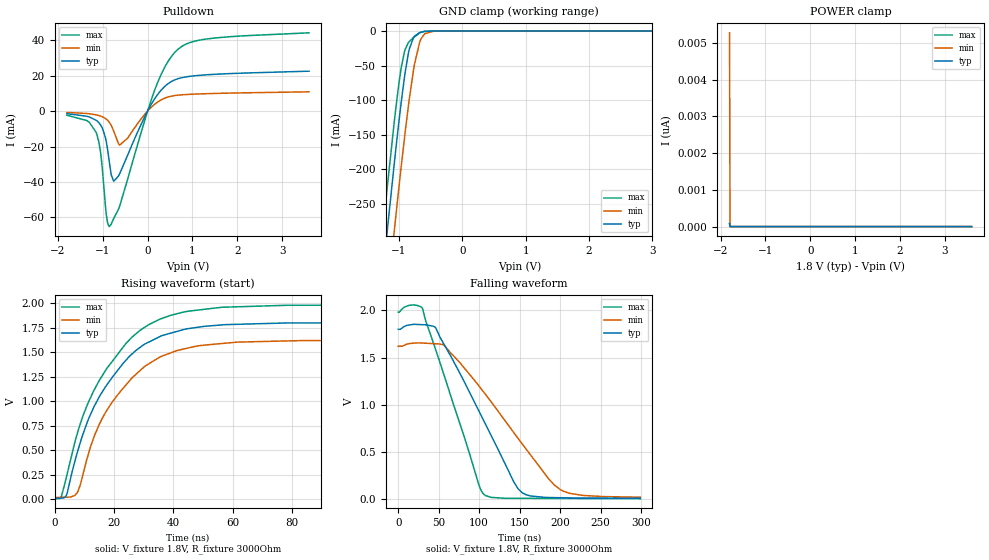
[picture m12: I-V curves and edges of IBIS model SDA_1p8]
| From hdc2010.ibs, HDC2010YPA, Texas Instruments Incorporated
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[Model]   SDA_1p8
Model_type   I/O_open_drain
Polarity   Non-Inverting
Enable   Active-Low
Vinl = 0.54
Vinh = 1.26
Vmeas = 0.9
Vref = 1.8
Cref = 15pF
Rref = 3000
|   typ   min   max
|   (nom PVT)   (slow PVT)   (fast PVT)
C_comp   1.615p   1.567p   1.665p
|C_comp (ON state)   1.615p   1.567p   1.665p
|C_comp (OFF state)   1.693p   1.643p   1.788p
[Model spec]
|subparameter
Vinl   0.54   0.486   0.594
Vinh   1.26   1.134   1.386
[Voltage Range]   1.8   1.62   1.98
[Temperature Range]   27   125   -40
[Pullup Reference]   1.8   1.62   1.98
[Pulldown Reference]   0   -0   0
[Power Clamp Reference]   1.8   1.62   1.98
[GND Clamp Reference]   0   0   0
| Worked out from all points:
|   slope of the pulldown table from 0 to 0.27 V, typ, clamps not added: 24.9 ohm
|   GND clamp passes 1 mA (typ) near -0.62 V on its own axis
|   falling waveform, V_fixture 1.8V, R_fixture 3000Ohm: 20-80 % time 62.9ns typ, 84.5ns min, 44.7ns max; typ from 1.8 V to 0.012 V
|   rising waveform, V_fixture 1.8V, R_fixture 3000Ohm: 20-80 % time 18.1ns typ, 18.1ns min, 18.6ns max; typ from 0.012 V to 1.8 V
[Pulldown]
|   Voltage   I(typ)   I(min)   I(max)
-1.8V     -1.437mA   -727.9uA   -2.321mA
-1.357V   -2.889mA   -1.337mA   -5.326mA
-1.147V   -5.182mA   -2.104mA   -12.02mA
-1.044V   -7.982mA   -2.835mA   -24.2mA
-941.4mV  -14.84mA   -4.15mA    -53.24mA
-855mV    -28.46mA   -6.275mA   -65.18mA
-757.8mV  -39.48mA   -11.11mA   -60.71mA
-622.8mV  -35.34mA   -19.16mA   -53.64mA
144mV     6.419mA    3.56mA     10.89mA
613.8mV   17.72mA    8.81mA     33.33mA
1.294V    20.47mA    9.831mA    40.63mA
3.6V      22.55mA    10.9mA     44.2mA
[GND Clamp]
|   Voltage   I(typ)   I(min)   I(max)
-1.8V     -872.1mA   -967.8mA   -810.9mA
-1.454V   -541.5mA   -639.3mA   -478.7mA
-1.222V   -325.5mA   -424.1mA   -262.4mA
-1.179V   -286.4mA   -385mA     -223.6mA
-1.071V   -191.5mA   -289mA     -131.1mA
-957.6mV  -99.89mA   -192.7mA   -50.89mA
-849.6mV  -32.61mA   -109.2mA   -16.94mA
-752.4mV  -7.509mA   -48.16mA   -8.453mA
-671.4mV  -2.23mA    -16.41mA   -2.849mA
-590.4mV  -477uA     -3.794mA   -452.8uA
-444.6mV  -11.28uA   -174.1uA   -3.034uA
3.6V      0A         0A         0A
[POWER Clamp]
|   Voltage   I(typ)   I(min)   I(max)
-1.8V     83.82pA    5.278nA    74.76pA
-1.789V   0A         0A         0A
-1.784V   0A         0A         0A
3.6V      0A         0A         0A
[Ramp]
R_load = 3000
|   typ   min   max
dV/dt_r   1.07306/1.81433e-08   0.960679/1.7943e-08   1.18357/1.86727e-08
dV/dt_f   1.0727/6.27864e-08   0.958128/8.41216e-08   1.18354/4.47004e-08
[Falling Waveform]
V_fixture = 1.8V
V_fixture_min = 1.62V
V_fixture_max = 1.98V
R_fixture = 3000Ohm
C_fixture = 0F
|   Time   V(typ)   V(min)   V(max)
0s        1.8V       1.62V      1.98V
29.84ns   1.849V     1.654V     2.024V
46.09ns   1.818V     1.647V     1.589V
57.3ns    1.63V      1.625V     1.297V
99.47ns   939.3mV    1.204V     158.8mV
106.5ns   819.4mV    1.126V     48.54mV
143.1ns   180.7mV    702.8mV    11.46mV
157.9ns   49.32mV    533.2mV    11.07mV
206.4ns   16.56mV    78.57mV    9.825mV
299ns     12.16mV    23.11mV    7.44mV
[Rising Waveform]
V_fixture = 1.8V
V_fixture_min = 1.62V
V_fixture_max = 1.98V
R_fixture = 3000Ohm
C_fixture = 0F
|   Time   V(typ)   V(min)   V(max)
0s        11.54mV    18.71mV    7.386mV
2.166ns   12.84mV    20.63mV    23.96mV
3.867ns   38.64mV    22.13mV    219.8mV
7.68ns    486.3mV    72.64mV    679mV
13.46ns   955.5mV    654.8mV    1.123V
17.52ns   1.164V     904.4mV    1.331V
28.75ns   1.547V     1.311V     1.72V
42.82ns   1.724V     1.526V     1.903V
83.19ns   1.797V     1.617V     1.977V
299ns     1.8V       1.62V      1.98V
